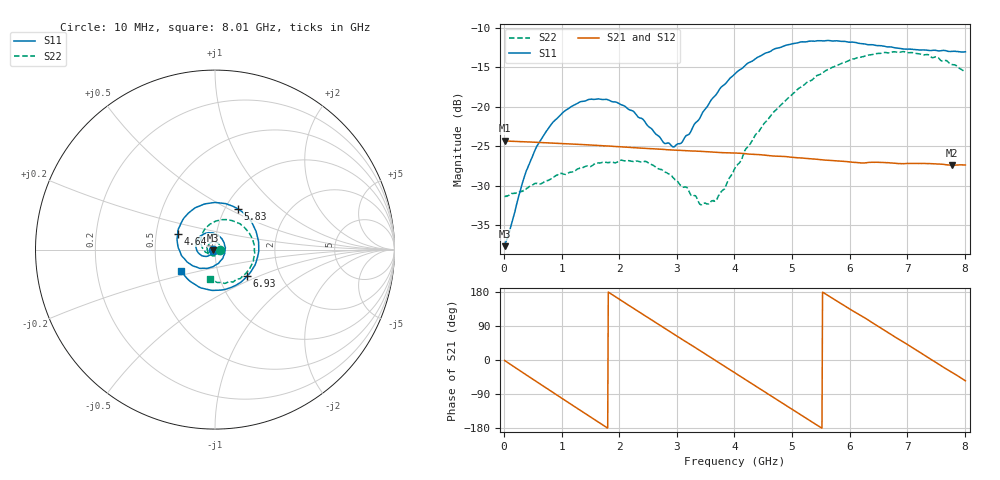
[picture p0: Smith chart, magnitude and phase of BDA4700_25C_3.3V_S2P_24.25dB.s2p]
!Agilent Technologies,E5071B,MY42404982,A.09.10
!Date: Mon Oct 20 18:13:15 2025
!Data & Calibration Information:
!Freq	S11:SOLT2(ON)	S21:SOLT2(ON)	S12:SOLT2(ON)	S22:SOLT2(ON)
# Hz S RI R 50
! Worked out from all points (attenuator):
!   801 points, 10 MHz to 8.01 GHz, reference 50 ohm
!   highest |S21| = -24.31 dB at 10 MHz (marker M1); lowest = -27.4 dB at 7.77 GHz (marker M2)
!   lowest |S11| = -37.7 dB at 10 MHz (marker M3), VSWR 1.03, Z = 48.7 - j0.141 ohm
!   |S11| at or under -10 dB: start of sweep to end of sweep
!   |S22| runs from -32.4 to -13.0 dB; largest |S21 - S12| = 0.0007
!   S11 on the Smith chart (normalised r, x): 10 MHz: 0.97, -0.00; 4.64 GHz: 0.65, +0.12; 5.83 GHz: 1.15, +0.56; 6.93 GHz: 1.36, -0.42; 8.01 GHz: 0.67, -0.17
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1e7  -0.013 -0.00145  0.0609 -0.0013  0.0608 -0.00134  0.0271 -0.000817
3.5e8  -0.0239 -0.0265  0.0487 -0.0349  0.0487 -0.0349  0.0229 -0.0184
5.8e8  -0.043 -0.0375  0.0309 -0.0508  0.0309 -0.0508  0.0144 -0.0292
1e9  -0.0871 -0.0241  -0.0107 -0.0575  -0.0107 -0.0575  -0.0146 -0.0349
1.35e9  -0.1069 0.0163  -0.041 -0.0404  -0.041 -0.0405  -0.0366 -0.0183
1.97e9  -0.056 0.09  -0.0536 0.016  -0.0536 0.016  -0.0348 0.028
2.45e9  0.0215 0.0768  -0.0243 0.0486  -0.0244 0.0487  -0.00319 0.045
2.68e9  0.0486 0.0437  -0.00403 0.0537  -0.0041 0.0537  0.0131 0.0383
2.97e9  0.055 -0.0124  0.0213 0.0485  0.0212 0.0485  0.0264 0.022
3.43e9  -0.00125 -0.0893  0.0484 0.0194  0.0484 0.0195  0.0201 -0.0131
3.69e9  -0.0606 -0.104  0.0513 -0.00287  0.0514 -0.00298  0.00139 -0.0255
4.01e9  -0.1403 -0.0799  0.0421 -0.0286  0.0421 -0.0285  -0.0313 -0.0261
4.64e9  -0.2078 0.0896  -0.00461 -0.0486  -0.00449 -0.0486  -0.0786 0.0406
4.97e9  -0.1621 0.1884  -0.029 -0.0382  -0.0289 -0.0384  -0.0679 0.0947
5.35e9  -0.0464 0.2561  -0.0449 -0.0131  -0.0448 -0.0134  -0.016 0.147
5.83e9  0.1279 0.2269  -0.0395 0.022  -0.0394 0.0221  0.0907 0.1625
6.26e9  0.2295 0.0992  -0.016 0.041  -0.0154 0.0412  0.1814 0.1034
6.68e9  0.2307 -0.0643  0.0144 0.0418  0.0145 0.0417  0.2196 -5.37e-05
6.93e9  0.179 -0.1478  0.0293 0.0322  0.0295 0.0321  0.2124 -0.0696
7.34e9  0.0378 -0.2248  0.0431 0.00656  0.0432 0.00665  0.1431 -0.1595
7.77e9  -0.1268 -0.1849  0.036 -0.0226  0.036 -0.0227  0.0282 -0.183
8.01e9  -0.1887 -0.1185  0.0246 -0.0349  0.0248 -0.035  -0.0301 -0.1631
